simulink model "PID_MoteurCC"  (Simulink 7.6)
settings: Solver=ode23t  StartTime=0.0  StopTime=0.6  RelTol=1e-3
InitFcn:
  | R1=1e3;
  | R2=10e3;
  | C1=1e-3;
  | C2=10e-3;
StopFcn:
  | clc
  | load consigne_position.mat
  | plotyy(x(1,:),x(2,:),x(1,:),x(3,:))
  | title('Régulateur PID - Signaux de commande et de vitesse de l''arbre moteur')
  | grid
  | %axis([0 1.5e-3 0 2])
  | xlabel('temps')
  | 
  | figure
  | plot(x(1,:),x(4,:),x(1,:),x(5,:))
  | title('Régulateur PID - Consigne et position de l''arbre moteur')
  | grid
  | %axis([0 1.5e-3 0 2])
  | xlabel('temps')
libraries: fl_lib x20, nesl_utility x5, elec_lib x2

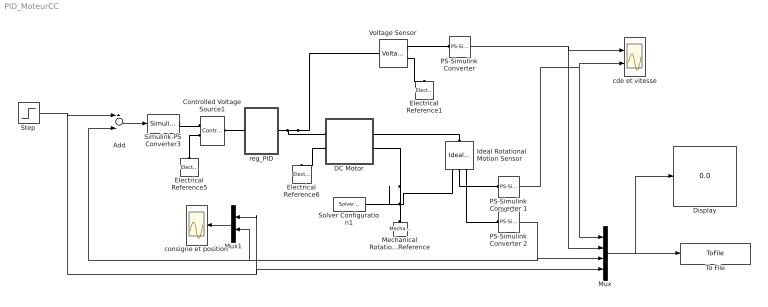
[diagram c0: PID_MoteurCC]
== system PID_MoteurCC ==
  Add : Sum  Inputs=+-
  Controlled Voltage Source1 : fl_lib/Electrical/Electrical Sources/Controlled Voltage Source  DialogController=NetworkEngine.DynNeDlgSource  SystemSampleTime=-1  i_Log=off  v_Log=off  LocalVarNames=|current|voltage|power  LocalVarDescs=|Current (A)|Voltage (V)|Power (W)  LocalVarLogging=[0 0 0]
  DC Motor : Subsystem
  Display : Display
  Electrical Reference1 : fl_lib/Electrical/Electrical Elements/Electrical Reference  DialogController=NetworkEngine.DynNeDlgSource  SystemSampleTime=-1  i_Log=off  LocalVarNames=|i  LocalVarDescs=|i  LocalVarLogging=[]
  Electrical Reference5 : fl_lib/Electrical/Electrical Elements/Electrical Reference  DialogController=NetworkEngine.DynNeDlgSource  SystemSampleTime=-1  i_Log=off  LocalVarNames=|i  LocalVarDescs=|i  LocalVarLogging=[]
  Electrical Reference6 : fl_lib/Electrical/Electrical Elements/Electrical Reference  DialogController=NetworkEngine.DynNeDlgSource  SystemSampleTime=-1  i_Log=off  LocalVarNames=|i  LocalVarDescs=|i  LocalVarLogging=[]
  Ideal Rotational Motion Sensor : fl_lib/Mechanical/Mechanical Sensors/Ideal Rotational Motion Sensor  DialogController=NetworkEngine.DynNeDlgSource  SystemSampleTime=-1  offset=0 rad  w_Log=off  t_Log=off  phi_Log=off  LocalVarNames=|w|t|phi  LocalVarDescs=|w|t|phi  LocalVarLogging=[]
  Mechanical Rotational Reference : fl_lib/Mechanical/Rotational Elements/Mechanical Rotational Reference  DialogController=NetworkEngine.DynNeDlgSource  SystemSampleTime=-1  t_Log=off  LocalVarNames=|t  LocalVarDescs=|t  LocalVarLogging=[]
  Mux : Mux
  Mux1 : Mux  Inputs=2
  PS-Simulink Converter : nesl_utility/PS-Simulink Converter  DialogController=NetworkEngine.DynNeUtilDlgSource  SystemSampleTime=-1  PhysicalDomain=network_engine_domain  LeftPortType=input  RightPortType=output  SubClassName=ps_output  Unit=1  AffineConversion=off
  PS-Simulink Converter 1 : nesl_utility/PS-Simulink Converter  DialogController=NetworkEngine.DynNeUtilDlgSource  SystemSampleTime=-1  PhysicalDomain=network_engine_domain  LeftPortType=input  RightPortType=output  SubClassName=ps_output  Unit=1  AffineConversion=off
  PS-Simulink Converter 2 : nesl_utility/PS-Simulink Converter  DialogController=NetworkEngine.DynNeUtilDlgSource  SystemSampleTime=-1  PhysicalDomain=network_engine_domain  LeftPortType=input  RightPortType=output  SubClassName=ps_output  Unit=1  AffineConversion=off
  Simulink-PS Converter3 : nesl_utility/Simulink-PS Converter  DialogController=NetworkEngine.DynNeUtilDlgSource  SystemSampleTime=-1  PhysicalDomain=network_engine_domain  LeftPortType=input  RightPortType=output  SubClassName=ps_input  Unit=1  AffineConversion=off  InputFilterTimeConstant=.001  UdotUserProvided=0
  Solver Configuration1 : nesl_utility/Solver Configuration  DialogController=NetworkEngine.DynNeUtilDlgSource  SystemSampleTime=-1  PhysicalDomain=network_engine_domain  LeftPortType=input  RightPortType=generic  SubClassName=solver  Accelerate=off  Profile=off  ResidualTolerance=1e-9  MaxNonlinIter=12  MaxModeIter=2  DoFixedCost=off  UseLocalSampling=off  DoDC=off  LinearAlgebra=Sparse  LocalSolverSampleTime=.001  LocalSolverChoice=NE_BACKWARD_EULER_ADVANCER  UseLocalSolver=off
  Step : Step  Time=0  After=100  SampleTime=0
  To File : ToFile  Filename=consigne_position  MatrixName=x
  Voltage Sensor : fl_lib/Electrical/Electrical Sensors/Voltage Sensor  DialogController=NetworkEngine.DynNeDlgSource  SystemSampleTime=-1  i1_Log=off  v1_Log=off  LocalVarNames=|i1|v1  LocalVarDescs=|i1|v1  LocalVarLogging=[0 0]
  cde et vitesse : Scope  NumInputPorts=2
  consigne et position : Scope
  reg_PID : Subsystem
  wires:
  PS-Simulink Converter 2/1 -> Mux/3, Add/2, Mux1/2
  Step/1 -> Add/1, Mux/4, Mux1/1
  Mux/1 -> To File/1, Display/1
  PS-Simulink Converter/1 -> cde et vitesse/1, Mux/2
  Add/1 -> Simulink-PS Converter3/1
  PS-Simulink Converter 1/1 -> cde et vitesse/2, Mux/1
  Mux1/1 -> consigne et position/1
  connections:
  Electrical Reference5/LConn1 -- Controlled Voltage Source1/RConn2
  Controlled Voltage Source1/LConn1 -- reg_PID/LConn1
  DC Motor/LConn2 -- Electrical Reference6/LConn1
  Voltage Sensor/RConn1 -- PS-Simulink Converter/LConn1
  Voltage Sensor/RConn2 -- Electrical Reference1/LConn1
  reg_PID/RConn1 -- Voltage Sensor/LConn1 -- DC Motor/LConn1
  Solver Configuration1/RConn1 -- DC Motor/RConn2 -- Mechanical Rotational Reference/LConn1 -- Ideal Rotational Motion Sensor/RConn1
  Simulink-PS Converter3/RConn1 -- Controlled Voltage Source1/RConn1
  Ideal Rotational Motion Sensor/LConn1 -- DC Motor/RConn1
  Ideal Rotational Motion Sensor/RConn3 -- PS-Simulink Converter 2/LConn1
  Ideal Rotational Motion Sensor/RConn2 -- PS-Simulink Converter 1/LConn1

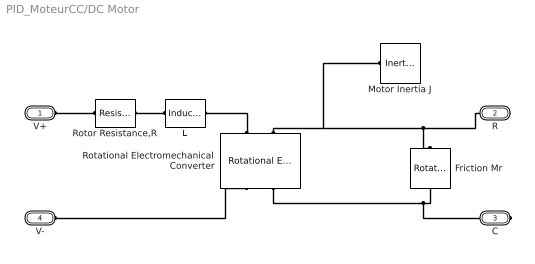
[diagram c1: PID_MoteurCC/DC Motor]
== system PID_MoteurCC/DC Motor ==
  Friction Mr : fl_lib/Mechanical/Rotational Elements/Rotational Friction  DialogController=NetworkEngine.DynNeDlgSource  SystemSampleTime=-1  brkwy_trq=0.02e-3 N*m  Col_trq=0.02e-3 N*m  visc_coef=0 N*m/(rad/s)  trans_coef=10 s/rad  vel_thr=0.1 rad/s  t_Log=off  w_Log=off  LocalVarNames=|friction_torque|rel_velocity|power  LocalVarDescs=|Friction torque (N*m)|Relative velocity (rad/s)|Power (W)  LocalVarLogging=[0 0 0]
  L : fl_lib/Electrical/Electrical Elements/Inductor  DialogController=NetworkEngine.DynNeDlgSource  SystemSampleTime=-1  l=12e-6 H  i0=0 A  r=0 Ohm  g=1e-09 1/Ohm  i_Log=off  v_Log=off  i_L_Log=off  LocalVarNames=|current|voltage|power  LocalVarDescs=|Inductor current (A) |Voltage across inductor (V)|Power (W)  LocalVarLogging=[0 0 0]
  Motor Inertia J : fl_lib/Mechanical/Rotational Elements/Inertia  DialogController=NetworkEngine.DynNeDlgSource  SystemSampleTime=-1  inertia=0.01 g*cm^2  initial_velocity=0 rad/s  t_Log=off  LocalVarNames=|torque|velocity  LocalVarDescs=|Inertia torque (N*m)|Inertia absolute velocity (rad/s)  LocalVarLogging=[0 0]
  Rotational Electromechanical Converter : fl_lib/Electrical/Electrical Elements/Rotational Electromechanical Converter  DialogController=NetworkEngine.DynNeDlgSource  SystemSampleTime=-1  K=0.072e-3*60/(2*pi) s*V/rad  i_Log=off  v_Log=off  t_Log=off  w_Log=off  LocalVarNames=|current|voltage|power|torque|speed  LocalVarDescs=|Current (A)|Voltage (V)|Power (W)|Torque (Nm)|Angular speed (rad/s)  LocalVarLogging=[0 0 0 0 0]
  Rotor Resistance,R : fl_lib/Electrical/Electrical Elements/Resistor  Tag=Factory Generic  DialogController=NetworkEngine.DynNeDlgSource  SystemSampleTime=-1  R=3.9 Ohm  i_Log=off  v_Log=off  LocalVarNames=|current|voltage|power  LocalVarDescs=|Resistor current (A)|Voltage across resistor (V)|Power (W)  LocalVarLogging=[0 0 0]
  V+ : PMIOPort  Port=1  Side=Left
  R : PMIOPort  Port=2  Side=Right
  C : PMIOPort  Port=3  Side=Right
  V- : PMIOPort  Port=4  Side=Left
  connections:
  Rotational Electromechanical Converter/LConn1 -- L/RConn1
  V-/RConn1 -- Rotational Electromechanical Converter/RConn1
  Rotor Resistance,R/LConn1 -- V+/RConn1
  L/LConn1 -- Rotor Resistance,R/RConn1
  Rotational Electromechanical Converter/LConn2 -- R/RConn1 -- Friction Mr/LConn1 -- Motor Inertia J/LConn1
  Rotational Electromechanical Converter/RConn2 -- C/RConn1 -- Friction Mr/RConn1

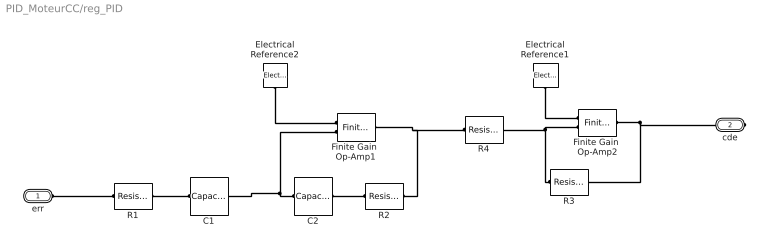
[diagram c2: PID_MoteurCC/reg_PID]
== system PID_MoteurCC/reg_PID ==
  C1 : fl_lib/Electrical/Electrical Elements/Capacitor  DialogController=NetworkEngine.DynNeDlgSource  SystemSampleTime=-1  c=C1 F  v0=0 V  r=1e-6 Ohm  g=0 1/Ohm  i_Log=off  v_Log=off  vc_Log=off  LocalVarNames=|i|v|vc  LocalVarDescs=|i|v|Internal variable for voltage across capacitor term  LocalVarLogging=[0 0 0]
  C2 : fl_lib/Electrical/Electrical Elements/Capacitor  DialogController=NetworkEngine.DynNeDlgSource  SystemSampleTime=-1  c=C2 F  v0=0 V  r=1e-6 Ohm  g=0 1/Ohm  i_Log=off  v_Log=off  vc_Log=off  LocalVarNames=|i|v|vc  LocalVarDescs=|i|v|Internal variable for voltage across capacitor term  LocalVarLogging=[0 0 0]
  Electrical Reference1 : fl_lib/Electrical/Electrical Elements/Electrical Reference  DialogController=NetworkEngine.DynNeDlgSource  SystemSampleTime=-1  i_Log=off  LocalVarNames=|i  LocalVarDescs=|i  LocalVarLogging=[]
  Electrical Reference2 : fl_lib/Electrical/Electrical Elements/Electrical Reference  DialogController=NetworkEngine.DynNeDlgSource  SystemSampleTime=-1  i_Log=off  LocalVarNames=|i  LocalVarDescs=|i  LocalVarLogging=[]
  Finite Gain  Op-Amp1 : elec_lib/Integrated Circuits/Finite Gain Op-Amp  DialogController=NetworkEngine.DynNeDlgSource  SystemSampleTime=-1  A=1000  Rin=1e+6 Ohm  Rout=100 Ohm  Vmin=-15 V  Vmax=15 V  LocalVarLogging=[]
  Finite Gain  Op-Amp2 : elec_lib/Integrated Circuits/Finite Gain Op-Amp  DialogController=NetworkEngine.DynNeDlgSource  SystemSampleTime=-1  A=1000  Rin=1e+6 Ohm  Rout=100 Ohm  Vmin=-15 V  Vmax=15 V  LocalVarLogging=[]
  R1 : fl_lib/Electrical/Electrical Elements/Resistor  DialogController=NetworkEngine.DynNeDlgSource  SystemSampleTime=-1  R=R1 Ohm  i_Log=off  v_Log=off  LocalVarNames=|current|voltage|power  LocalVarDescs=|Resistor current (A)|Voltage across resistor (V)|Power (W)  LocalVarLogging=[0 0 0]
  R2 : fl_lib/Electrical/Electrical Elements/Resistor  DialogController=NetworkEngine.DynNeDlgSource  SystemSampleTime=-1  R=R2 Ohm  i_Log=off  v_Log=off  LocalVarNames=|current|voltage|power  LocalVarDescs=|Resistor current (A)|Voltage across resistor (V)|Power (W)  LocalVarLogging=[0 0 0]
  R3 : fl_lib/Electrical/Electrical Elements/Resistor  DialogController=NetworkEngine.DynNeDlgSource  SystemSampleTime=-1  R=R2 Ohm  i_Log=off  v_Log=off  LocalVarNames=|current|voltage|power  LocalVarDescs=|Resistor current (A)|Voltage across resistor (V)|Power (W)  LocalVarLogging=[0 0 0]
  R4 : fl_lib/Electrical/Electrical Elements/Resistor  DialogController=NetworkEngine.DynNeDlgSource  SystemSampleTime=-1  R=R2 Ohm  i_Log=off  v_Log=off  LocalVarNames=|current|voltage|power  LocalVarDescs=|Resistor current (A)|Voltage across resistor (V)|Power (W)  LocalVarLogging=[0 0 0]
  err : PMIOPort  Port=1  Side=Left
  cde : PMIOPort  Port=2  Side=Right
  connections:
  R3/LConn1 -- Finite Gain  Op-Amp2/LConn2 -- R4/RConn1
  Finite Gain  Op-Amp1/LConn2 -- C2/LConn1 -- C1/RConn1
  C2/RConn1 -- R2/LConn1
  R1/LConn1 -- err/RConn1
  Electrical Reference2/LConn1 -- Finite Gain  Op-Amp1/LConn1
  C1/LConn1 -- R1/RConn1
  Finite Gain  Op-Amp2/RConn1 -- cde/RConn1 -- R3/RConn1
  R2/RConn1 -- Finite Gain  Op-Amp1/RConn1 -- R4/LConn1
  Electrical Reference1/LConn1 -- Finite Gain  Op-Amp2/LConn1
